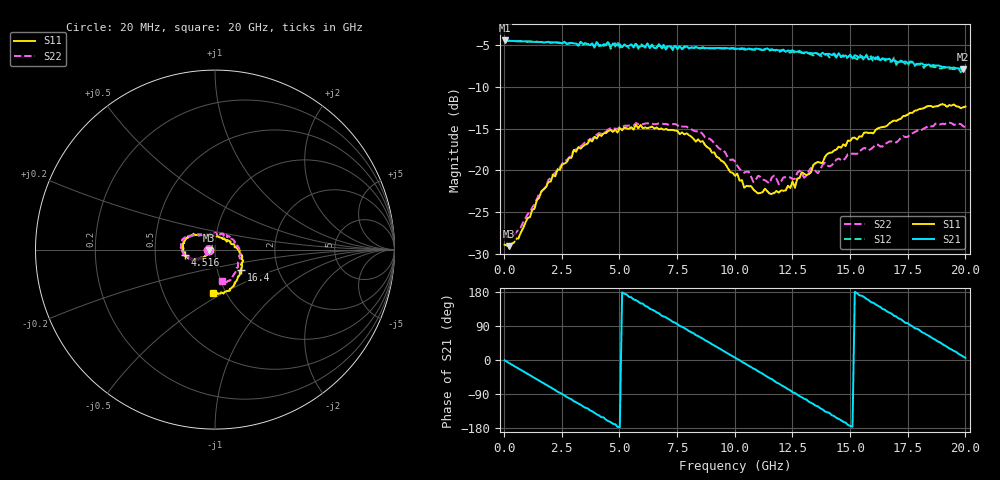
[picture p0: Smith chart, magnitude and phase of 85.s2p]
!Agilent Technologies,N5230A,US43500223,A.07.50.48
!Agilent N5230A: A.07.50.48
!Date: Saturday, October 10, 2015 17:45:36
!Correction: S11(Full 2 Port(1,2))
!S21(Full 2 Port(1,2))
!S12(Full 2 Port(1,2))
!S22(Full 2 Port(1,2))
!S2P File: Measurements: S11, S21, S12, S22:
# Hz S  RI  R 50
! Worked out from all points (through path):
!   201 points, 20 MHz to 20 GHz, reference 50 ohm
!   highest |S21| = -4.44 dB at 20 MHz (marker M1); lowest = -7.9 dB at 19.9 GHz (marker M2)
!   group delay of S21, straight-line fit = 99 ps
!   lowest |S11| = -29.1 dB at 219.8 MHz (marker M3), VSWR 1.07, Z = 46.6 - j0.386 ohm
!   |S11| at or under -10 dB: start of sweep to end of sweep
!   |S22| runs from -28.1 to -14.3 dB; largest |S21 - S12| = 0.033
!   S11 on the Smith chart (normalised r, x): 20 MHz: 0.93, +0.00; 4.516 GHz: 0.71, -0.04; 16.4 GHz: 1.30, -0.30; 20 GHz: 0.87, -0.45
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2e7  -0.0359 0.000274  0.6 -0.0083  0.599 -0.00751  -0.0403 3.33e-05
2.198e8  -0.0349 -0.00414  0.591 -0.0852  0.5911 -0.0856  -0.0399 -0.00329
1.9181e9  -0.0685 -0.0507  0.2113 -0.55  0.2099 -0.548  -0.0755 -0.0444
2.6174e9  -0.0937 -0.0573  -0.034 -0.589  -0.0332 -0.5807  -0.1033 -0.0495
3.4166e9  -0.1296 -0.0519  -0.3049 -0.4823  -0.3131 -0.4714  -0.1336 -0.0505
4.5155e9  -0.1699 -0.029  -0.5539 -0.1863  -0.5658 -0.184  -0.1737 -0.0293
5.7143e9  -0.188 0.00752  -0.5313 0.2157  -0.5385 0.2178  -0.1917 0.0114
6.7133e9  -0.1719 0.039  -0.3124 0.477  -0.3081 0.4724  -0.1873 0.0383
7.4126e9  -0.1613 0.0624  -0.0829 0.5507  -0.087 0.5542  -0.1803 0.0585
8.3117e9  -0.1257 0.0794  0.2261 0.5004  0.2241 0.4879  -0.1574 0.0679
1.001e10  -0.0457 0.0806  0.5332 0.0566  0.5298 0.0553  -0.0799 0.08
1.09091e10  -0.00467 0.0745  0.4848 -0.2284  0.4739 -0.2305  -0.0306 0.0823
1.18082e10  0.035 0.0666  0.2663 -0.4556  0.2654 -0.4457  0.00966 0.0885
1.25075e10  0.0676 0.0531  0.0439 -0.5221  0.0454 -0.5127  0.0278 0.0841
1.34066e10  0.1034 0.0298  -0.2202 -0.4511  -0.2035 -0.4428  0.0695 0.0759
1.4006e10  0.1251 0.00622  -0.3707 -0.3352  -0.374 -0.3232  0.0897 0.0581
1.5005e10  0.1475 -0.0284  -0.4901 -0.0516  -0.4832 -0.0691  0.1217 0.0306
1.64036e10  0.1438 -0.1112  -0.328 0.3305  -0.3407 0.3238  0.1337 -0.0377
1.67033e10  0.1407 -0.1291  -0.2662 0.3825  -0.2611 0.3622  0.1375 -0.0573
1.83017e10  0.0839 -0.2256  0.163 0.3916  0.157 0.4014  0.0965 -0.1533
1.99001e10  -0.00517 -0.2382  0.3982 0.0643  0.3964 0.0644  0.0414 -0.1793
2e10  -0.01 -0.2409  0.4059 0.0414  0.3985 0.0423  0.0411 -0.176
